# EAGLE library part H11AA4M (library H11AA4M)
None Check prices
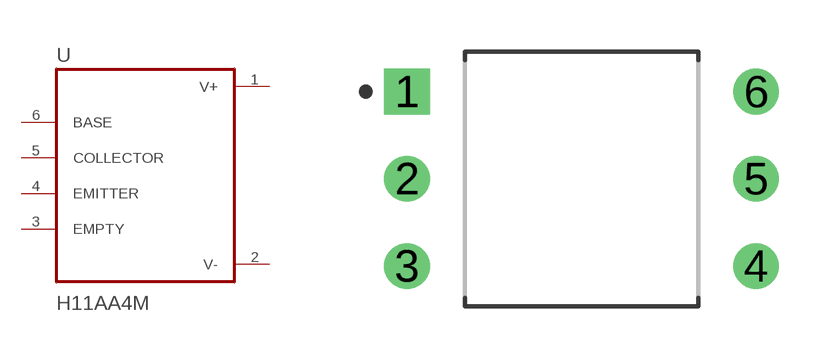
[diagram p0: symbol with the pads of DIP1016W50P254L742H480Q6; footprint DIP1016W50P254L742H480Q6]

Designator prefix U

## H11AA4M (Availability: Good; Description: AC-IN 1-CH Transistor With Base DC-OUT 6-Pin PDIP Bag; MF: ON Semiconductor; MP: H11AA4M; Package: PDIP-6 ON Semiconductor; Price: None; Purchase-URL: https://pricing.snapeda.com/search/part/H11AA4M/?ref=eda)  [DIP1016W50P254L742H480Q6]
1  V+  pwr
2  V-  pwr
3  EMPTY
4  EMITTER
5  COLLECTOR
6  BASE

## Footprint DIP1016W50P254L742H480Q6 (pad centres in mm)
Optocoupler DC Input 1 Channel Trans W/Base DC Output 6-Pin Plastic Dip White
drill 0.82 square: 1 -5.08,2.54
drill 0.82: 2 -5.08,0; 3 -5.08,-2.54; 4 5.08,-2.54; 5 5.08,0; 6 5.08,2.54

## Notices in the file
This work is licensed under a Creative Commons Attribution-ShareAlike 4.0 International License (CC BY-SA) with Design Exception 1.0
